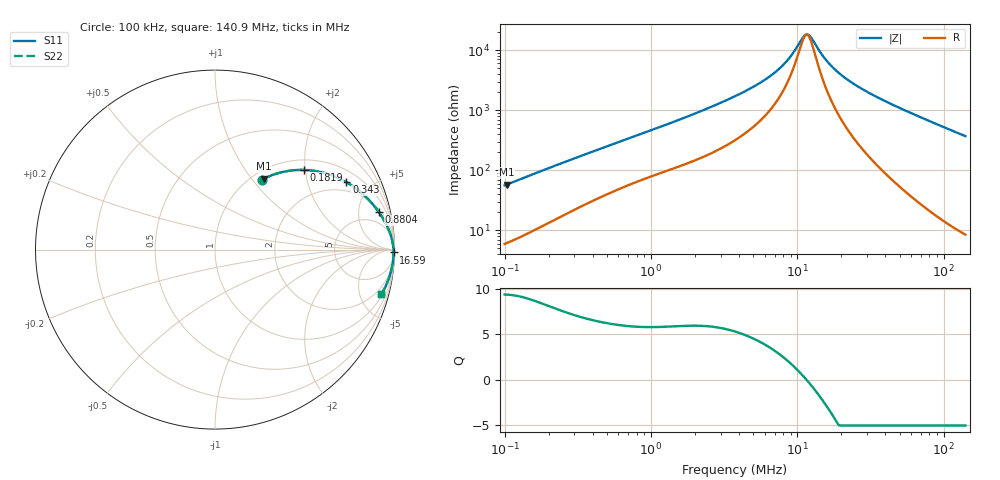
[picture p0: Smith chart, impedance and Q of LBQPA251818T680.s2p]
! LBQPA251818T680  S-PARAMETER MODEL  ( General Type )
! Model Generated by TAIYO YUDEN Corporation (http://www.ty-top.com)
! Version 1.0
! TAIYO YUDEN Control No. 191025NI43SB-FBB
! Copyright(c) 2019 TAIYO YUDEN CO.,LTD. All Rights Reserved.
! Product Description (link to TY-COMPAS)
! https://ds.yuden.co.jp/TYCOMPAS/or/detail?pn=LBQPA251818T680K&u=M
! Products Name : Inductors
! Characteristics :
!  Inductance : 68 uH , SRF(min) : 9.5 MHz , DC Resistance(max) : 3.64 Ohm
!  Rated Current : Saturation :200 mA , Temp Rise : 140 mA (20 degC)
!  Case Size : 2.5 x 1.8 / 0.098 x 0.071 [mm/inch] , Thickness : 1.8 / 0.071 [mm/inch]
!  (Conditions: Temperature = 25 degC , DC Bias Current/Voltage = 0A / 0V)
! External Node Assignments :
!  1  o---GGG---o  2
! GND o---------o GND
! Frequency Range : 0.1MHz  -  140.89697MHz  [ 402 STEP ]
# MHz S RI R 50
! Freq[MHz].  S11 Real  S11 Imag  S21 Real  S21 Imag  S12 Real  S12 Imag  S22 Real  S22 Imag
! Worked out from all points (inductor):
!   401 points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, 100 kHz to 140.9 MHz, reference 50 ohm
!   read as one part in series: L = 87.8 uH near 103.7 kHz
!   highest Q = 9.35 at 103.7 kHz (marker M1), where L = 88.5 uH
!   self-resonance near 11.55 MHz
!   S11 on the Smith chart (normalised r, x): 100 kHz: 1.12, +1.11; 181.9 kHz: 1.24, +1.97; 343 kHz: 1.52, +3.53; 880.4 kHz: 2.40, +8.14; 16.59 MHz: open; 140.9 MHz: 1.17, -7.39
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0.1  0.2601 0.3885  0.7399 -0.3885  0.7399 -0.3885  0.2601 0.3885
0.103692  0.2724 0.395  0.7276 -0.395  0.7276 -0.395  0.2724 0.395
0.18188  0.4972 0.4437  0.5028 -0.4437  0.5028 -0.4437  0.4972 0.4437
0.336853  0.727 0.3786  0.273 -0.3786  0.273 -0.3786  0.727 0.3786
0.343015  0.7324 0.3755  0.2676 -0.3755  0.2676 -0.3755  0.7324 0.3755
0.529965  0.8382 0.2958  0.1618 -0.2958  0.1618 -0.2958  0.8382 0.2958
0.880381  0.9126 0.2091  0.0874 -0.2091  0.0874 -0.2091  0.9126 0.2091
1.134703  0.9366 0.1724  0.0634 -0.1724  0.0634 -0.1724  0.9366 0.1724
3.753625  0.9861 0.0561  0.0139 -0.0561  0.0139 -0.0561  0.9861 0.0561
5.492476  0.9906 0.0342  0.00936 -0.0342  0.00936 -0.0342  0.9906 0.0342
7.340476  0.9928 0.0201  0.00724 -0.0201  0.00724 -0.0201  0.9928 0.0201
8.799273  0.9937 0.012  0.00633 -0.012  0.00633 -0.012  0.9937 0.012
11.34118  0.9945 0.000928  0.00549 -0.000928  0.00549 -0.000928  0.9945 0.000928
11.97499  0.9946 -0.00144  0.00537 0.00144  0.00537 0.00144  0.9946 -0.00144
12.64421  0.9947 -0.00382  0.00528 0.00382  0.00528 0.00382  0.9947 -0.00382
14.61739  0.9949 -0.0103  0.00512 0.0103  0.00512 0.0103  0.9949 -0.0103
16.59494  0.9949 -0.0161  0.0051 0.0161  0.0051 0.0161  0.9949 -0.0161
19.53556  0.9948 -0.0241  0.00525 0.0241  0.00525 0.0241  0.9948 -0.0241
23.84629  0.9943 -0.0347  0.00573 0.0347  0.00573 0.0347  0.9943 -0.0347
42.59248  0.9899 -0.075  0.0101 0.075  0.0101 0.075  0.9899 -0.075
78.88411  0.9738 -0.1445  0.0262 0.1445  0.0262 0.1445  0.9738 -0.1445
140.897  0.9268 -0.2492  0.0732 0.2492  0.0732 0.2492  0.9268 -0.2492
